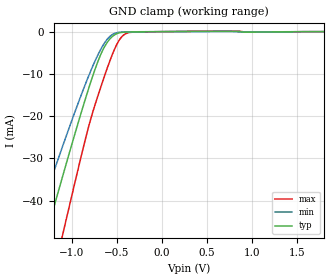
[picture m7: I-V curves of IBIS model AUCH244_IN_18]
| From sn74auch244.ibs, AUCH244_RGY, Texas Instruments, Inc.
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[Model]   AUCH244_IN_18
Model_type  Input
Vinl=0.5775
Vinh=1.2675
| variable   typ   min   max
C_comp   2.48pF   1.96pF   2.80pF
[Temperature Range]   40   100   -40
| Ambient temperature   25   85   -40
[Voltage range]   1.8   1.65   1.95
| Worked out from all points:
|   GND clamp passes 1 mA (typ) near -0.54 V on its own axis
[GND Clamp]
| AUCH244_IN_18
|   Voltage   I(typ)   I(min)   I(max)
-3.6V     -227.9mA   -191.3mA   -273.5mA
-1.435V   -59.52mA   -47.82mA   -78.45mA
-1.39V    -56.07mA   -44.96mA   -74.34mA
-1.26V    -46.14mA   -36.81mA   -62.48mA
-1.1V     -34.08mA   -26.98mA   -47.89mA
-1.055V   -30.74mA   -24.28mA   -43.79mA
-820mV    -13.93mA   -10.87mA   -23.03mA
-685mV    -5.734mA   -4.448mA   -13.57mA
-565mV    -1.467mA   -921.6uA   -6.238mA
-485mV    -373.1uA   -197.6uA   -2.435mA
-420mV    -128.2uA   -73.2uA    -731.9uA
1.8V      215.9pA    557.8nA    -950.7pA
